FUNCTION_BLOCK FB_PushPopStack
VAR_IN_OUT
	ArrayStmaterial: ARRAY[1..INUM] OF DUT_material;
END_VAR
VAR_INPUT
	PushStmaterial:  DUT_material;
END_VAR
VAR_OUTPUT
	PopStmaterial	: DUT_material;
	busy						: BOOL;
END_VAR
VAR
	i: INT;
END_VAR

;

METHOD PopStack : BOOL
VAR_INPUT
END_VAR

VAR
	i: INT;
END_VAR
busy:=TRUE;
PopStmaterial:=ArrayStmaterial[1];
FOR i:=2 TO INUM DO
	ArrayStmaterial[i-1]:=ArrayStmaterial[i];
END_FOR
ArrayStmaterial[INUM].bmaterial:=FALSE;
ArrayStmaterial[INUM].lrAngle:=0.0;
ArrayStmaterial[INUM].lrCenterX:=0.0;
ArrayStmaterial[INUM].lrCenterY:=0.0;
ArrayStmaterial[INUM].lrHeight:=0.0;
ArrayStmaterial[INUM].lrLength:=0.0;
ArrayStmaterial[INUM].lrPhotoBeltPos:=0.0;
ArrayStmaterial[INUM].lrPhotoTime:=0.0;
ArrayStmaterial[INUM].lrWidth:=0.0;
busy:=FALSE;
END_METHOD

METHOD PushStack : BOOL
VAR_INPUT
END_VAR
busy:=TRUE;
FOR i:=1 TO INUM DO
	IF NOT ArrayStmaterial[i].bmaterial THEN
		ArrayStmaterial[i]:=PushStmaterial;
		EXIT;
	END_IF
END_FOR
busy:=FALSE;
END_METHOD

END_FUNCTION_BLOCK
